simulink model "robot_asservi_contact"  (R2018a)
settings: Solver=VariableStepAuto  StartTime=0.0  StopTime=t(numel(t))  FixedStep=0.0001  RelTol=1e-3
model workspace: external: MATLAB File (data not in the file)
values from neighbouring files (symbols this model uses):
  D = [1500 1500 1000 0 0 0]    [TP_6Axes_main.m]
  dt = 0.01    [TP_6axes_trajectoire_polynomiale.m]    (also in TP_6axes_trajectoire_rectangulaire.m = 0.005)
  I = [0 0 0 0 0 0]    [TP_6Axes_main.m]
  mu = mu/3    [TP_6Axes_main.m]
  nx = length(ref)    [Jnum.m]    (also in TP_6axes_trajectoire_rectangulaire.m = 0.6)
  P = [16000 15000 14000 3000 3000 3000]    [TP_6Axes_main.m]
  q_targ = zeros(6,numel(p_targ(1,:)))    [TP_6axes_trajectoire_polynomiale.m]    (also in TP_6axes_trajectoire_rectangulaire.m)
  X = [T(1:3,4);Euler]    [MGD_6axes.m]    (also in TP_6axes_trajectoire_polynomiale.m = Trace_6axes_trajectoire(q_targ,p_targ,rob); TP_6axes_trajectoire_rectangulaire.m = Trace_6axes_trajectoire(q_targ,p_targ,rob); Trace_6axes.m = [0 0 0; Trace_6axes_trajectoire.m = [0 0 0)
undefined symbols (not defined in the file or in its folder): deg, kg, m, mm, N, rad, s, smiData, Y, Z
libraries: sm_lib x42, nesl_utility x23, Contact_Forces_Lib x1
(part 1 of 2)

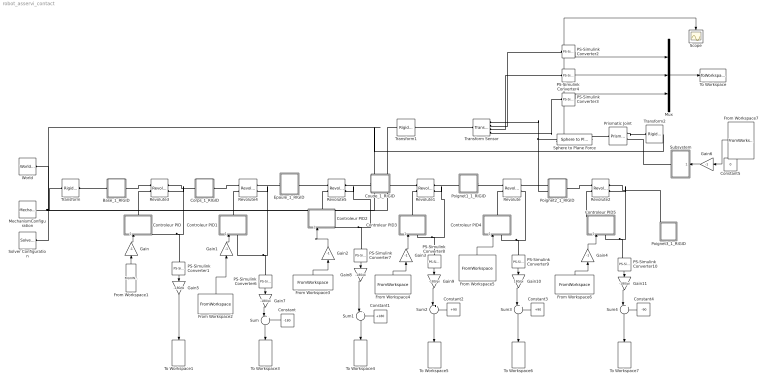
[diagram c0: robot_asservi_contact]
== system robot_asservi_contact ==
  Base_1_RIGID : Subsystem
  Constant : Constant  Value=-180
  Constant1 : Constant  Value=+180
  Constant2 : Constant  Value=+90
  Constant3 : Constant  Value=+90
  Constant4 : Constant  Value=-90
  Constant5 : Constant  Value=0
  Controleur PID : Subsystem
  Controleur PID1 : Subsystem
  Controleur PID2 : Subsystem
  Controleur PID3 : Subsystem
  Controleur PID4 : Subsystem
  Controleur PID5 : Subsystem
  Corps_1_RIGID : Subsystem
  Coude_1_RIGID : Subsystem
  Epaule_1_RIGID : Subsystem
  From Workspace1 : FromWorkspace  VariableName=[t' q_targ(1,:)']  SampleTime=0
  From Workspace2 : FromWorkspace  VariableName=[t' q_targ(2,:)'+pi]  SampleTime=0
  From Workspace3 : FromWorkspace  VariableName=[t' q_targ(3,:)'-pi]  SampleTime=0
  From Workspace4 : FromWorkspace  VariableName=[t' q_targ(4,:)'-pi/2]  SampleTime=0
  From Workspace5 : FromWorkspace  VariableName=[t' q_targ(5,:)'-pi/2]  SampleTime=0
  From Workspace6 : FromWorkspace  VariableName=[t' q_targ(6,:)'+pi/2]  SampleTime=0
  From Workspace7 : FromWorkspace  VariableName=[t' delta'];
  Gain{,1..4,6} (6 alike) : Gain  Gain=-1
  Gain10 : Gain  Gain=180/pi
  Gain{5,7..9,11} (5 alike) : Gain  Gain=-180/pi
  MechanismConfiguration : sm_lib/Utilities/Mechanism Configuration  UniformGravity=None  GravityVector=[0 -9.80665 0]  GravityUnits=m/s^2  LinearizationDelta=0.001
  Mux : Mux  Inputs=3
  PS-Simulink Converter{1,6..10} (6 alike) : nesl_utility/PS-Simulink Converter  PhysicalDomain=network_engine_domain  SubClassName=ps_output  LeftPortType=input  RightPortType=output  PseudoPeriodic=off  Frequencies=[]  Unit=rad  AffineConversion=off
  PS-Simulink Converter2 : nesl_utility/PS-Simulink Converter  PhysicalDomain=network_engine_domain  SubClassName=ps_output  LeftPortType=input  RightPortType=output  PseudoPeriodic=off  Frequencies=[]  Unit=1  AffineConversion=off
  PS-Simulink Converter3 : nesl_utility/PS-Simulink Converter  PhysicalDomain=network_engine_domain  SubClassName=ps_output  LeftPortType=input  RightPortType=output  PseudoPeriodic=off  Frequencies=[]  Unit=1  AffineConversion=off
  PS-Simulink Converter4 : nesl_utility/PS-Simulink Converter  PhysicalDomain=network_engine_domain  SubClassName=ps_output  LeftPortType=input  RightPortType=output  PseudoPeriodic=off  Frequencies=[]  Unit=1  AffineConversion=off
  Poignet1_1_RIGID : Subsystem
  Poignet2_1_RIGID : Subsystem
  Poignet3_1_RIGID : Subsystem
  Prismatic Joint : sm_lib/Joints/Prismatic Joint  SenseConstraintForce=off  SenseConstraintForceX=off  SenseConstraintForceY=off  SenseConstraintForceZ=off  SenseConstraintTorque=off  SenseConstraintTorqueX=off  SenseConstraintTorqueY=off  SenseConstraintTorqueZ=off  SenseTotalForce=off  SenseTotalForceX=off  SenseTotalForceY=off  SenseTotalForceZ=off  SenseTotalTorque=off  SenseTotalTorqueX=off  SenseTotalTorqueY=off  SenseTotalTorqueZ=off  CompositeWrenchDir=FollowerOnBase  CompositeWrenchFrame=BaseFrame  EquilibriumPosition=0  EquilibriumPositionUnits=m  SpringStiffness=0  SpringStiffnessUnits=N/m  DampingCoefficient=0  DampingCoefficientUnits=N/(m/s)  TorqueActuationMode=ComputedTorque  MotionActuationMode=InputMotion  SensePosition=off  SenseVelocity=off  SenseAcceleration=off  SenseTorqueForce=off  PositionTargetSpecify=off  PositionTargetPriority=High  PositionTargetValue=0  PositionTargetValueUnits=m  VelocityTargetSpecify=off  VelocityTargetPriority=High  VelocityTargetValue=0  VelocityTargetValueUnits=m/s
  Revolute : sm_lib/Joints/Revolute Joint  SenseConstraintForce=off  SenseConstraintForceX=off  SenseConstraintForceY=off  SenseConstraintForceZ=off  SenseConstraintTorque=off  SenseConstraintTorqueX=off  SenseConstraintTorqueY=off  SenseConstraintTorqueZ=off  SenseTotalForce=off  SenseTotalForceX=off  SenseTotalForceY=off  SenseTotalForceZ=off  SenseTotalTorque=off  SenseTotalTorqueX=off  SenseTotalTorqueY=off  SenseTotalTorqueZ=off  CompositeWrenchDir=FollowerOnBase  CompositeWrenchFrame=BaseFrame  EquilibriumPosition=0  EquilibriumPositionUnits=rad  SpringStiffness=0  SpringStiffnessUnits=N*m/rad  DampingCoefficient=1/mu(5)  DampingCoefficientUnits=N*m/(rad/s)  TorqueActuationMode=InputTorque  MotionActuationMode=ComputedMotion  SensePosition=on  SenseVelocity=off  SenseAcceleration=off  SenseTorqueForce=off  PositionTargetSpecify=on  PositionTargetPriority=High  PositionTargetValue=q_targ(5,1)-pi/2  PositionTargetValueUnits=rad  VelocityTargetSpecify=off  VelocityTargetPriority=High  VelocityTargetValue=0  VelocityTargetValueUnits=deg/s
  Revolute1 : sm_lib/Joints/Revolute Joint  SenseConstraintForce=off  SenseConstraintForceX=off  SenseConstraintForceY=off  SenseConstraintForceZ=off  SenseConstraintTorque=off  SenseConstraintTorqueX=off  SenseConstraintTorqueY=off  SenseConstraintTorqueZ=off  SenseTotalForce=off  SenseTotalForceX=off  SenseTotalForceY=off  SenseTotalForceZ=off  SenseTotalTorque=off  SenseTotalTorqueX=off  SenseTotalTorqueY=off  SenseTotalTorqueZ=off  CompositeWrenchDir=FollowerOnBase  CompositeWrenchFrame=BaseFrame  EquilibriumPosition=0  EquilibriumPositionUnits=rad  SpringStiffness=0  SpringStiffnessUnits=N*m/rad  DampingCoefficient=1/mu(4)  DampingCoefficientUnits=N*m/(rad/s)  TorqueActuationMode=InputTorque  MotionActuationMode=ComputedMotion  SensePosition=on  SenseVelocity=off  SenseAcceleration=off  SenseTorqueForce=off  PositionTargetSpecify=on  PositionTargetPriority=High  PositionTargetValue=-q_targ(4,1)+pi/2  PositionTargetValueUnits=rad  VelocityTargetSpecify=off  VelocityTargetPriority=High  VelocityTargetValue=0  VelocityTargetValueUnits=deg/s
  Revolute2 : sm_lib/Joints/Revolute Joint  SenseConstraintForce=off  SenseConstraintForceX=off  SenseConstraintForceY=off  SenseConstraintForceZ=off  SenseConstraintTorque=off  SenseConstraintTorqueX=off  SenseConstraintTorqueY=off  SenseConstraintTorqueZ=off  SenseTotalForce=off  SenseTotalForceX=off  SenseTotalForceY=off  SenseTotalForceZ=off  SenseTotalTorque=off  SenseTotalTorqueX=off  SenseTotalTorqueY=off  SenseTotalTorqueZ=off  CompositeWrenchDir=FollowerOnBase  CompositeWrenchFrame=BaseFrame  EquilibriumPosition=0  EquilibriumPositionUnits=rad  SpringStiffness=0  SpringStiffnessUnits=N*m/rad  DampingCoefficient=1/mu(6)  DampingCoefficientUnits=N*m/(rad/s)  TorqueActuationMode=InputTorque  MotionActuationMode=ComputedMotion  SensePosition=on  SenseVelocity=off  SenseAcceleration=off  SenseTorqueForce=off  PositionTargetSpecify=on  PositionTargetPriority=High  PositionTargetValue=-q_targ(6,1)-pi/2  PositionTargetValueUnits=rad  VelocityTargetSpecify=off  VelocityTargetPriority=High  VelocityTargetValue=0  VelocityTargetValueUnits=deg/s
  Revolute3 : sm_lib/Joints/Revolute Joint  SenseConstraintForce=off  SenseConstraintForceX=off  SenseConstraintForceY=off  SenseConstraintForceZ=off  SenseConstraintTorque=off  SenseConstraintTorqueX=off  SenseConstraintTorqueY=off  SenseConstraintTorqueZ=off  SenseTotalForce=off  SenseTotalForceX=off  SenseTotalForceY=off  SenseTotalForceZ=off  SenseTotalTorque=off  SenseTotalTorqueX=off  SenseTotalTorqueY=off  SenseTotalTorqueZ=off  CompositeWrenchDir=FollowerOnBase  CompositeWrenchFrame=BaseFrame  EquilibriumPosition=0  EquilibriumPositionUnits=rad  SpringStiffness=0  SpringStiffnessUnits=N*m/rad  DampingCoefficient=1/mu(1)  DampingCoefficientUnits=N*m/(rad/s)  TorqueActuationMode=InputTorque  MotionActuationMode=ComputedMotion  SensePosition=on  SenseVelocity=off  SenseAcceleration=off  SenseTorqueForce=off  PositionTargetSpecify=on  PositionTargetPriority=High  PositionTargetValue=-q_targ(1,1)  PositionTargetValueUnits=rad  VelocityTargetSpecify=off  VelocityTargetPriority=High  VelocityTargetValue=0  VelocityTargetValueUnits=deg/s
  Revolute4 : sm_lib/Joints/Revolute Joint  SenseConstraintForce=off  SenseConstraintForceX=off  SenseConstraintForceY=off  SenseConstraintForceZ=off  SenseConstraintTorque=off  SenseConstraintTorqueX=off  SenseConstraintTorqueY=off  SenseConstraintTorqueZ=off  SenseTotalForce=off  SenseTotalForceX=off  SenseTotalForceY=off  SenseTotalForceZ=off  SenseTotalTorque=off  SenseTotalTorqueX=off  SenseTotalTorqueY=off  SenseTotalTorqueZ=off  CompositeWrenchDir=FollowerOnBase  CompositeWrenchFrame=BaseFrame  EquilibriumPosition=0  EquilibriumPositionUnits=rad  SpringStiffness=0  SpringStiffnessUnits=N*m/rad  DampingCoefficient=1/mu(2)  DampingCoefficientUnits=N*m/(rad/s)  TorqueActuationMode=InputTorque  MotionActuationMode=ComputedMotion  SensePosition=on  SenseVelocity=off  SenseAcceleration=off  SenseTorqueForce=off  PositionTargetSpecify=on  PositionTargetPriority=High  PositionTargetValue=-q_targ(2,1)-pi  PositionTargetValueUnits=rad  VelocityTargetSpecify=off  VelocityTargetPriority=High  VelocityTargetValue=0  VelocityTargetValueUnits=deg/s
  Revolute5 : sm_lib/Joints/Revolute Joint  SenseConstraintForce=off  SenseConstraintForceX=off  SenseConstraintForceY=off  SenseConstraintForceZ=off  SenseConstraintTorque=off  SenseConstraintTorqueX=off  SenseConstraintTorqueY=off  SenseConstraintTorqueZ=off  SenseTotalForce=off  SenseTotalForceX=off  SenseTotalForceY=off  SenseTotalForceZ=off  SenseTotalTorque=off  SenseTotalTorqueX=off  SenseTotalTorqueY=off  SenseTotalTorqueZ=off  CompositeWrenchDir=FollowerOnBase  CompositeWrenchFrame=BaseFrame  EquilibriumPosition=0  EquilibriumPositionUnits=rad  SpringStiffness=0  SpringStiffnessUnits=N*m/rad  DampingCoefficient=1/mu(3)  DampingCoefficientUnits=N*m/(rad/s)  TorqueActuationMode=InputTorque  MotionActuationMode=ComputedMotion  SensePosition=on  SenseVelocity=off  SenseAcceleration=off  SenseTorqueForce=off  PositionTargetSpecify=on  PositionTargetPriority=High  PositionTargetValue=-q_targ(3,1)+pi  PositionTargetValueUnits=rad  VelocityTargetSpecify=off  VelocityTargetPriority=High  VelocityTargetValue=0  VelocityTargetValueUnits=deg/s
  Scope : Scope
  Solver Configuration : nesl_utility/Solver Configuration  PhysicalDomain=network_engine_domain  SubClassName=solver  LeftPortType=input  RightPortType=generic  Tones=[]  Harmonics=[]  SimulateNoise=off  Profile=off  UseLocalSampling=off  EnableSwitchedLinearOptims=on  FrequencyDomain=off  UseCCode=off  RelTol=0.001  AbsTol=1e-06  MinStep=1e-09  ToWorkspace=off  RevertToSquareIcSolve=off  NumHomotopyIterations=100  PhasorMode=off  PhasorModeNumHarmonics=1  DoDC=off  ResidualTolerance=1e-09  UseLocalSolver=off  LocalSolverChoice=NE_BACKWARD_EULER_ADVANCER  LocalSolverSampleTime=0.001  DoFixedCost=off  MaxNonlinIter=3  MaxModeIter=2  LinearAlgebra=Sparse  EquationFormulation=NE_TIME_EF  DelaysMemoryBudget=1024  AutomaticFiltering=on  FilteringTimeConstant=0.001
  Sphere to Plane Force : Contact_Forces_Lib/3D/Sphere to Plane Force  sphere_rad=e/2  plane_lenx=1  plane_leny=1  plane_depth=e/2  force_law=Nonlinear  k_contact=1e4  b_contact=1e1  pen_full_damp_F=1e-4  pen_exponent=1  custom_param_1=1  custom_param_2=1  friction_law=None  mu_kinetic=0.5  mu_static=0.7  v_thr=0.001  vis_on=on  vis_opc_en=0  vis_len_plaBz=0.005  vis_clr=[0.9 0.2 0.2]  vis_opc=0.7
  Subsystem : Subsystem
  Sum{,1..4} (5 alike) : Sum  Inputs=|++
  To Workspace : ToWorkspace  VariableName=pos_poignet  SaveFormat=Structure  SampleTime=-1
  To Workspace1 : ToWorkspace  VariableName=q_real1  SampleTime=dt
  To Workspace3 : ToWorkspace  VariableName=q_real2  SampleTime=dt
  To Workspace4 : ToWorkspace  VariableName=q_real3  SampleTime=dt
  To Workspace5 : ToWorkspace  VariableName=q_real4  SampleTime=dt
  To Workspace6 : ToWorkspace  VariableName=q_real5  SampleTime=dt
  To Workspace7 : ToWorkspace  VariableName=q_real6  SampleTime=dt
  Transform : sm_lib/Frames and Transforms/Rigid Transform  TranslationMethod=Cartesian  TranslationStandardOffset=0  TranslationLengthUnit=mm  TranslationStandardAxis=+Z  TranslationCartesianOffset=smiData.RigidTransform(10).translation  TranslationROffset=0  TranslationROffsetUnits=m  TranslationZOffset=0  TranslationZOffsetUnits=m  TranslationThetaOffset=0  TranslationThetaOffsetUnits=deg  RotationMethod=ArbitraryAxis  RotationAngleUnits=rad  RotationStandardAxis=+Z  RotationAngle=smiData.RigidTransform(10).angle  RotationArbitraryAxis=smiData.RigidTransform(10).axis  FollAlignAxisA=+X  BaseAlignAxisA=+Y  FollAlignAxisB=+Y  BaseAlignAxisB=+Z  RotationSequenceAxes=FollowerAxes  RotationSequence=XYX  RotationSequenceAngles=[0 0 0]  RotationSequenceAnglesUnits=deg  RotationMatrix=[1 0 0; 0 1 0; 0 0 1]
  Transform Sensor : sm_lib/Frames and Transforms/Transform Sensor  MeasurementFrame=World  SenseAngle=off  SenseAxis=off  SenseAngle1=off  SenseAngle2=off  SenseAngle3=off  SenseQ=off  SenseR=off  SenseOmegaX=off  SenseOmegaY=off  SenseOmegaZ=off  SenseOmega1=off  SenseOmega2=off  SenseOmega3=off  SenseQDot=off  SenseRDot=off  SenseAlphaX=off  SenseAlphaY=off  SenseAlphaZ=off  SenseAlpha1=off  SenseAlpha2=off  SenseAlpha3=off  SenseQDDot=off  SenseRDDot=off  SenseX=on  SenseY=on  SenseZ=on  SenseRad=off  SenseAzim=off  SenseDist=off  SenseInc=off  SenseXDot=off  SenseYDot=off  SenseZDot=off  SenseRadDot=off  SenseAzimDot=off  SenseDistDot=off  SenseIncDot=off  SenseXDDot=off  SenseYDDot=off  SenseZDDot=off  SenseRadDDot=off  SenseAzimDDot=off  SenseDistDDot=off  SenseIncDDot=off
  Transform1 : sm_lib/Frames and Transforms/Rigid Transform  TranslationMethod=StandardAxis  TranslationStandardOffset=350  TranslationLengthUnit=mm  TranslationStandardAxis=+Z  TranslationCartesianOffset=smiData.RigidTransform(10).translation  TranslationROffset=0  TranslationROffsetUnits=m  TranslationZOffset=0  TranslationZOffsetUnits=m  TranslationThetaOffset=0  TranslationThetaOffsetUnits=deg  RotationMethod=None  RotationAngleUnits=rad  RotationStandardAxis=+Z  RotationAngle=smiData.RigidTransform(10).angle  RotationArbitraryAxis=smiData.RigidTransform(10).axis  FollAlignAxisA=+X  BaseAlignAxisA=+Y  FollAlignAxisB=+Y  BaseAlignAxisB=+Z  RotationSequenceAxes=FollowerAxes  RotationSequence=XYX  RotationSequenceAngles=[0 0 0]  RotationSequenceAnglesUnits=deg  RotationMatrix=[1 0 0; 0 1 0; 0 0 1]
  Transform2 : sm_lib/Frames and Transforms/Rigid Transform  TranslationMethod=Cartesian  TranslationStandardOffset=350  TranslationLengthUnit=m  TranslationStandardAxis=+Z  TranslationCartesianOffset=[nx+e/2 0 0.35]  TranslationROffset=0  TranslationROffsetUnits=m  TranslationZOffset=0  TranslationZOffsetUnits=m  TranslationThetaOffset=0  TranslationThetaOffsetUnits=deg  RotationMethod=StandardAxis  RotationAngleUnits=rad  RotationStandardAxis=+Y  RotationAngle=-pi/2  RotationArbitraryAxis=smiData.RigidTransform(10).axis  FollAlignAxisA=+X  BaseAlignAxisA=+Y  FollAlignAxisB=+Y  BaseAlignAxisB=+Z  RotationSequenceAxes=FollowerAxes  RotationSequence=XYX  RotationSequenceAngles=[0 0 0]  RotationSequenceAnglesUnits=deg  RotationMatrix=[1 0 0; 0 1 0; 0 0 1]
  World : sm_lib/Frames and Transforms/World Frame
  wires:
  PS-Simulink Converter2/1 -> Mux/1
  PS-Simulink Converter3/1 -> Mux/3
  PS-Simulink Converter4/1 -> Mux/2
  Mux/1 -> To Workspace/1
  From Workspace2/1 -> Gain1/1
  From Workspace1/1 -> Gain/1
  From Workspace6/1 -> Gain4/1
  Gain/1 -> Controleur PID/1(consigne)
  From Workspace3/1 -> Gain2/1
  Gain1/1 -> Controleur PID1/1(consigne)
  From Workspace4/1 -> Gain3/1
  Gain4/1 -> Controleur PID5/1(consigne)
  From Workspace5/1 -> Controleur PID4/1(consigne)
  Gain2/1 -> Controleur PID2/1(consigne)
  Gain3/1 -> Controleur PID3/1(consigne)
  PS-Simulink Converter1/1 -> Gain5/1
  Gain5/1 -> To Workspace1/1
  PS-Simulink Converter6/1 -> Gain7/1
  PS-Simulink Converter7/1 -> Gain8/1
  PS-Simulink Converter8/1 -> Gain9/1
  PS-Simulink Converter9/1 -> Gain10/1
  PS-Simulink Converter10/1 -> Gain11/1
  Gain7/1 -> Sum/1
  Sum/1 -> To Workspace3/1
  Gain9/1 -> Sum2/1
  Gain11/1 -> Sum4/1
  Gain10/1 -> Sum3/1
  Gain8/1 -> Sum1/1
  Sum1/1 -> To Workspace4/1
  Sum2/1 -> To Workspace5/1
  Sum3/1 -> To Workspace6/1
  Sum4/1 -> To Workspace7/1
  Constant/1 -> Sum/2
  Constant1/1 -> Sum1/2
  Constant2/1 -> Sum2/2
  Constant3/1 -> Sum3/2
  Constant4/1 -> Sum4/2
  Sphere to Plane Force/1 -> Scope/1
  Gain6/1 -> Subsystem/1(In1)
  From Workspace7/1 -> Gain6/1
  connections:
  MechanismConfiguration/RConn1 -- Solver Configuration/RConn1 -- World/RConn1 -- Transform2/LConn1 -- Transform1/LConn1 -- Transform/LConn1
  Poignet1_1_RIGID/RConn1 -- Revolute/LConn1
  Corps_1_RIGID/RConn1 -- Revolute4/LConn1
  Epaule_1_RIGID/LConn1 -- Revolute4/RConn1
  Epaule_1_RIGID/RConn1 -- Revolute5/LConn1
  Coude_1_RIGID/LConn1 -- Revolute5/RConn1
  Poignet2_1_RIGID/LConn1 -- Revolute/RConn1
  Coude_1_RIGID/RConn1 -- Revolute1/LConn1
  Poignet1_1_RIGID/LConn1 -- Revolute1/RConn1
  Poignet2_1_RIGID/RConn1 -- Revolute2/LConn1
  Poignet3_1_RIGID/LConn1 -- Revolute2/RConn1
  Base_1_RIGID/RConn1 -- Revolute3/LConn1
  Corps_1_RIGID/LConn1 -- Revolute3/RConn1
  Base_1_RIGID/LConn1 -- Transform/RConn1
  PS-Simulink Converter3/LConn1 -- Transform Sensor/RConn4
  PS-Simulink Converter2/LConn1 -- Transform Sensor/RConn2
  Poignet2_1_RIGID/LConn2 -- Sphere to Plane Force/LConn1 -- Transform Sensor/RConn1
  Transform1/RConn1 -- Transform Sensor/LConn1
  Transform Sensor/RConn3 -- PS-Simulink Converter4/LConn1
  Controleur PID/RConn1 -- Revolute3/LConn2
  Controleur PID1/RConn1 -- Revolute4/LConn2
  Controleur PID5/RConn1 -- Revolute2/LConn2
  Controleur PID5/LConn1 -- PS-Simulink Converter10/LConn1 -- Revolute2/RConn2
  Controleur PID3/LConn1 -- PS-Simulink Converter8/LConn1 -- Revolute1/RConn2
  Controleur PID4/RConn1 -- Revolute/LConn2
  Controleur PID2/RConn1 -- Revolute5/LConn2
  Controleur PID2/LConn1 -- PS-Simulink Converter7/LConn1 -- Revolute5/RConn2
  Controleur PID3/RConn1 -- Revolute1/LConn2
  Controleur PID1/LConn1 -- PS-Simulink Converter6/LConn1 -- Revolute4/RConn2
  Controleur PID4/LConn1 -- PS-Simulink Converter9/LConn1 -- Revolute/RConn2
  Controleur PID/LConn1 -- PS-Simulink Converter1/LConn1 -- Revolute3/RConn2
  Sphere to Plane Force/RConn1 -- Prismatic Joint/RConn1
  Prismatic Joint/LConn1 -- Transform2/RConn1
  Subsystem/RConn1 -- Prismatic Joint/LConn2

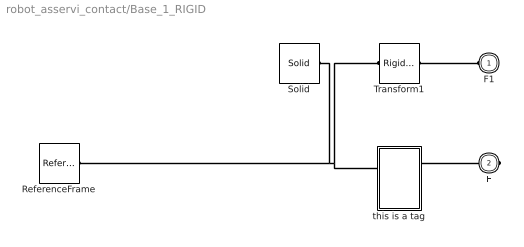
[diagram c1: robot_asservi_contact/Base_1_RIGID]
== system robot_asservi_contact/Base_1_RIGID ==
  ReferenceFrame : sm_lib/Frames and Transforms/Reference Frame
  Solid : sm_lib/Body Elements/Solid  InertiaType=Custom  Mass=smiData.Solid(1).mass  MassUnits=kg  CenterOfMass=smiData.Solid(1).CoM  CenterOfMassUnits=mm  MomentsOfInertia=smiData.Solid(1).MoI  MomentsOfInertiaUnits=kg*mm^2  ProductsOfInertia=smiData.Solid(1).PoI  ProductsOfInertiaUnits=kg*mm^2  DensityBased=on  Density=1000  DensityUnits=kg/m^3  DoExposeReferenceFrame=on  SerializedFrames=<Frames/>  GraphicType=FromGeometry  MarkerShape=Sphere  MarkerSize=10  GraphicVisPropType=SimpleVisualProperties  GraphicDiffuseColor=[1.0 0.0 0.0]  GraphicSpecularColor=[0.5 0.5 0.5 1.0]  GraphicAmbientColor=[0.15 0.15 0.15 1.0]  GraphicEmissiveColor=[0.0 0.0 0.0 1.0]  GraphicShininess=75  GraphicOpacity=smiData.Solid(1).opacity  GeometryShape=FromFile  RectangleSize=[1 1]  RectangleSizeUnits=m  BrickDimensions=[1 1 1]  BrickDimensionUnits=m  CylinderRadius=1  CylinderRadiusUnits=m  CylinderLength=1  CylinderLengthUnits=m  SphereRadius=1  SphereRadiusUnits=m  EllipsoidRadii=[1 1 1]  EllipsoidRadiiUnits=m  ExtrusionCrossSection=[1 1; -1 1; -1 -1; 1 -1]  ExtrusionCrossSectionUnits=m  ExtrusionLength=1  ExtrusionLengthUnits=m  PolygonNumSides=3  PolygonOuterRadius=1  PolygonOuterRadiusUnits=m  ExtGeomFileType=STL  ExtGeomFileName=Base_Défaut_sldprt.STL  ExtGeomFileUnits=mm  RevolutionCrossSection=[1 1; 1 -1; 2 -1; 2 1]  RevolutionCrossSectionUnits=m  RevolutionExtent=Full  RevolutionAngle=180  RevolutionAngleUnits=deg
  Transform1 : sm_lib/Frames and Transforms/Rigid Transform  TranslationMethod=Cartesian  TranslationStandardOffset=0  TranslationLengthUnit=mm  TranslationStandardAxis=+Z  TranslationCartesianOffset=smiData.RigidTransform(9).translation  TranslationROffset=0  TranslationROffsetUnits=m  TranslationZOffset=0  TranslationZOffsetUnits=m  TranslationThetaOffset=0  TranslationThetaOffsetUnits=deg  RotationMethod=ArbitraryAxis  RotationAngleUnits=rad  RotationStandardAxis=+Z  RotationAngle=smiData.RigidTransform(9).angle  RotationArbitraryAxis=smiData.RigidTransform(9).axis  FollAlignAxisA=+X  BaseAlignAxisA=+Y  FollAlignAxisB=+Y  BaseAlignAxisB=+Z  RotationSequenceAxes=FollowerAxes  RotationSequence=XYX  RotationSequenceAngles=[0 0 0]  RotationSequenceAnglesUnits=deg  RotationMatrix=[1 0 0; 0 1 0; 0 0 1]
  this is a tag : Subsystem
  F1 : PMIOPort  Side=Left
  F : PMIOPort  Port=2  Side=Right
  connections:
  Transform1/RConn1 -- F1/RConn1
  ReferenceFrame/RConn1 -- Solid/RConn1 -- this is a tag/LConn1 -- Transform1/LConn1
  this is a tag/RConn1 -- F/RConn1

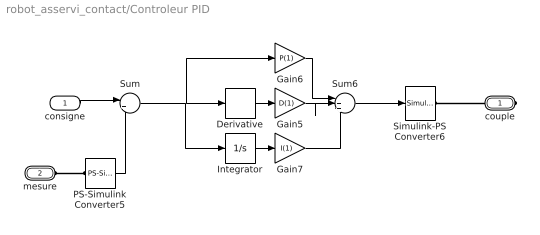
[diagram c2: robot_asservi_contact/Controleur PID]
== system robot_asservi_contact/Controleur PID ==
  consigne : Inport
  Derivative : Derivative
  Gain5 : Gain  Gain=D(1)
  Gain6 : Gain  Gain=P(1)
  Gain7 : Gain  Gain=I(1)
  Integrator : Integrator
  PS-Simulink Converter5 : nesl_utility/PS-Simulink Converter  PhysicalDomain=network_engine_domain  SubClassName=ps_output  LeftPortType=input  RightPortType=output  PseudoPeriodic=off  Frequencies=[]  Unit=rad  AffineConversion=off
  Simulink-PS Converter6 : nesl_utility/Simulink-PS Converter  PhysicalDomain=network_engine_domain  SubClassName=ps_input  LeftPortType=input  RightPortType=output  PseudoPeriodic=off  Frequencies=[]  NoiseDistribution=none  NoiseParameters=[]  Unit=N*m  AffineConversion=off  FilteringAndDerivatives=zero  SimscapeFilterOrder=1  InputFilterTimeConstant=0.001  UdotUserProvided=2
  Sum : Sum  Inputs=|+-
  Sum6 : Sum  Inputs=|+++
  couple : PMIOPort  Side=Right
  mesure : PMIOPort  Port=2  Side=Left
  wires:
  Gain7/1 -> Sum6/3
  Gain5/1 -> Sum6/2
  Derivative/1 -> Gain5/1
  Sum6/1 -> Simulink-PS Converter6/1
  Gain6/1 -> Sum6/1
  Integrator/1 -> Gain7/1
  consigne/1 -> Sum/1
  PS-Simulink Converter5/1 -> Sum/2
  Sum/1 -> Integrator/1, Gain6/1, Derivative/1
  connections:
  Simulink-PS Converter6/RConn1 -- couple/RConn1
  mesure/RConn1 -- PS-Simulink Converter5/LConn1

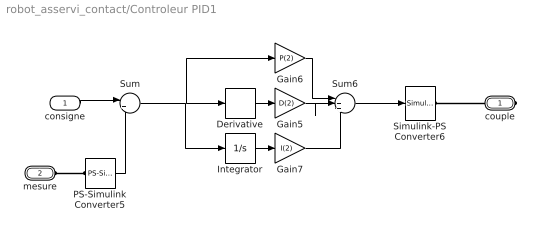
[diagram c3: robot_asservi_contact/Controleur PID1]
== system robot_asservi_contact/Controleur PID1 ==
  consigne : Inport
  Derivative : Derivative
  Gain5 : Gain  Gain=D(2)
  Gain6 : Gain  Gain=P(2)
  Gain7 : Gain  Gain=I(2)
  Integrator : Integrator
  PS-Simulink Converter5 : nesl_utility/PS-Simulink Converter  PhysicalDomain=network_engine_domain  SubClassName=ps_output  LeftPortType=input  RightPortType=output  PseudoPeriodic=off  Frequencies=[]  Unit=rad  AffineConversion=off
  Simulink-PS Converter6 : nesl_utility/Simulink-PS Converter  PhysicalDomain=network_engine_domain  SubClassName=ps_input  LeftPortType=input  RightPortType=output  PseudoPeriodic=off  Frequencies=[]  NoiseDistribution=none  NoiseParameters=[]  Unit=N*m  AffineConversion=off  FilteringAndDerivatives=zero  SimscapeFilterOrder=1  InputFilterTimeConstant=0.001  UdotUserProvided=2
  Sum : Sum  Inputs=|+-
  Sum6 : Sum  Inputs=|+++
  couple : PMIOPort  Side=Right
  mesure : PMIOPort  Port=2  Side=Left
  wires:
  Gain7/1 -> Sum6/3
  Gain5/1 -> Sum6/2
  Derivative/1 -> Gain5/1
  Sum6/1 -> Simulink-PS Converter6/1
  Gain6/1 -> Sum6/1
  Integrator/1 -> Gain7/1
  consigne/1 -> Sum/1
  PS-Simulink Converter5/1 -> Sum/2
  Sum/1 -> Integrator/1, Gain6/1, Derivative/1
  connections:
  Simulink-PS Converter6/RConn1 -- couple/RConn1
  mesure/RConn1 -- PS-Simulink Converter5/LConn1

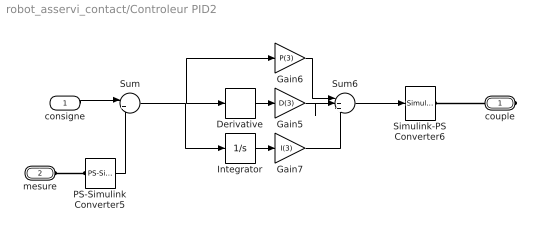
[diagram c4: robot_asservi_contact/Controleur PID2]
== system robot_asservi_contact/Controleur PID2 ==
  consigne : Inport
  Derivative : Derivative
  Gain5 : Gain  Gain=D(3)
  Gain6 : Gain  Gain=P(3)
  Gain7 : Gain  Gain=I(3)
  Integrator : Integrator
  PS-Simulink Converter5 : nesl_utility/PS-Simulink Converter  PhysicalDomain=network_engine_domain  SubClassName=ps_output  LeftPortType=input  RightPortType=output  PseudoPeriodic=off  Frequencies=[]  Unit=rad  AffineConversion=off
  Simulink-PS Converter6 : nesl_utility/Simulink-PS Converter  PhysicalDomain=network_engine_domain  SubClassName=ps_input  LeftPortType=input  RightPortType=output  PseudoPeriodic=off  Frequencies=[]  NoiseDistribution=none  NoiseParameters=[]  Unit=N*m  AffineConversion=off  FilteringAndDerivatives=zero  SimscapeFilterOrder=1  InputFilterTimeConstant=0.001  UdotUserProvided=2
  Sum : Sum  Inputs=|+-
  Sum6 : Sum  Inputs=|+++
  couple : PMIOPort  Side=Right
  mesure : PMIOPort  Port=2  Side=Left
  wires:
  Gain7/1 -> Sum6/3
  Gain5/1 -> Sum6/2
  Derivative/1 -> Gain5/1
  Sum6/1 -> Simulink-PS Converter6/1
  Gain6/1 -> Sum6/1
  Integrator/1 -> Gain7/1
  consigne/1 -> Sum/1
  PS-Simulink Converter5/1 -> Sum/2
  Sum/1 -> Integrator/1, Gain6/1, Derivative/1
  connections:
  Simulink-PS Converter6/RConn1 -- couple/RConn1
  mesure/RConn1 -- PS-Simulink Converter5/LConn1

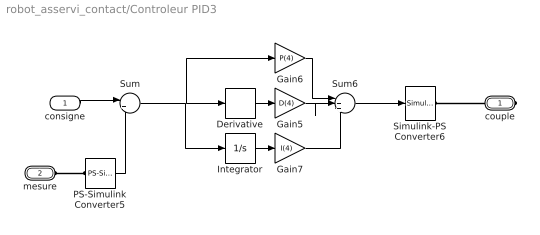
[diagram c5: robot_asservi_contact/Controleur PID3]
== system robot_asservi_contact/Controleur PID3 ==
  consigne : Inport
  Derivative : Derivative
  Gain5 : Gain  Gain=D(4)
  Gain6 : Gain  Gain=P(4)
  Gain7 : Gain  Gain=I(4)
  Integrator : Integrator
  PS-Simulink Converter5 : nesl_utility/PS-Simulink Converter  PhysicalDomain=network_engine_domain  SubClassName=ps_output  LeftPortType=input  RightPortType=output  PseudoPeriodic=off  Frequencies=[]  Unit=rad  AffineConversion=off
  Simulink-PS Converter6 : nesl_utility/Simulink-PS Converter  PhysicalDomain=network_engine_domain  SubClassName=ps_input  LeftPortType=input  RightPortType=output  PseudoPeriodic=off  Frequencies=[]  NoiseDistribution=none  NoiseParameters=[]  Unit=N*m  AffineConversion=off  FilteringAndDerivatives=zero  SimscapeFilterOrder=1  InputFilterTimeConstant=0.001  UdotUserProvided=2
  Sum : Sum  Inputs=|+-
  Sum6 : Sum  Inputs=|+++
  couple : PMIOPort  Side=Right
  mesure : PMIOPort  Port=2  Side=Left
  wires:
  Gain7/1 -> Sum6/3
  Gain5/1 -> Sum6/2
  Derivative/1 -> Gain5/1
  Sum6/1 -> Simulink-PS Converter6/1
  Gain6/1 -> Sum6/1
  Integrator/1 -> Gain7/1
  consigne/1 -> Sum/1
  PS-Simulink Converter5/1 -> Sum/2
  Sum/1 -> Integrator/1, Gain6/1, Derivative/1
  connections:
  Simulink-PS Converter6/RConn1 -- couple/RConn1
  mesure/RConn1 -- PS-Simulink Converter5/LConn1

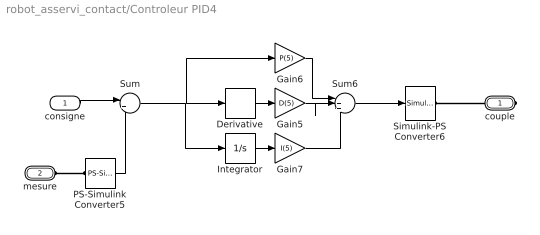
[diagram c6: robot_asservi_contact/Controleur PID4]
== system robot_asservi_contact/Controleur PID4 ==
  consigne : Inport
  Derivative : Derivative
  Gain5 : Gain  Gain=D(5)
  Gain6 : Gain  Gain=P(5)
  Gain7 : Gain  Gain=I(5)
  Integrator : Integrator
  PS-Simulink Converter5 : nesl_utility/PS-Simulink Converter  PhysicalDomain=network_engine_domain  SubClassName=ps_output  LeftPortType=input  RightPortType=output  PseudoPeriodic=off  Frequencies=[]  Unit=rad  AffineConversion=off
  Simulink-PS Converter6 : nesl_utility/Simulink-PS Converter  PhysicalDomain=network_engine_domain  SubClassName=ps_input  LeftPortType=input  RightPortType=output  PseudoPeriodic=off  Frequencies=[]  NoiseDistribution=none  NoiseParameters=[]  Unit=N*m  AffineConversion=off  FilteringAndDerivatives=zero  SimscapeFilterOrder=1  InputFilterTimeConstant=0.001  UdotUserProvided=2
  Sum : Sum  Inputs=|+-
  Sum6 : Sum  Inputs=|+++
  couple : PMIOPort  Side=Right
  mesure : PMIOPort  Port=2  Side=Left
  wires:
  Gain7/1 -> Sum6/3
  Gain5/1 -> Sum6/2
  Derivative/1 -> Gain5/1
  Sum6/1 -> Simulink-PS Converter6/1
  Gain6/1 -> Sum6/1
  Integrator/1 -> Gain7/1
  consigne/1 -> Sum/1
  PS-Simulink Converter5/1 -> Sum/2
  Sum/1 -> Integrator/1, Gain6/1, Derivative/1
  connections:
  Simulink-PS Converter6/RConn1 -- couple/RConn1
  mesure/RConn1 -- PS-Simulink Converter5/LConn1

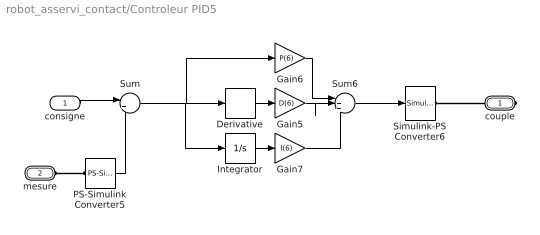
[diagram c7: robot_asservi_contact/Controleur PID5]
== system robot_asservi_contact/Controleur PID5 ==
  consigne : Inport
  Derivative : Derivative
  Gain5 : Gain  Gain=D(6)
  Gain6 : Gain  Gain=P(6)
  Gain7 : Gain  Gain=I(6)
  Integrator : Integrator
  PS-Simulink Converter5 : nesl_utility/PS-Simulink Converter  PhysicalDomain=network_engine_domain  SubClassName=ps_output  LeftPortType=input  RightPortType=output  PseudoPeriodic=off  Frequencies=[]  Unit=rad  AffineConversion=off
  Simulink-PS Converter6 : nesl_utility/Simulink-PS Converter  PhysicalDomain=network_engine_domain  SubClassName=ps_input  LeftPortType=input  RightPortType=output  PseudoPeriodic=off  Frequencies=[]  NoiseDistribution=none  NoiseParameters=[]  Unit=N*m  AffineConversion=off  FilteringAndDerivatives=zero  SimscapeFilterOrder=1  InputFilterTimeConstant=0.001  UdotUserProvided=2
  Sum : Sum  Inputs=|+-
  Sum6 : Sum  Inputs=|+++
  couple : PMIOPort  Side=Right
  mesure : PMIOPort  Port=2  Side=Left
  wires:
  Gain7/1 -> Sum6/3
  Gain5/1 -> Sum6/2
  Derivative/1 -> Gain5/1
  Sum6/1 -> Simulink-PS Converter6/1
  Gain6/1 -> Sum6/1
  Integrator/1 -> Gain7/1
  consigne/1 -> Sum/1
  PS-Simulink Converter5/1 -> Sum/2
  Sum/1 -> Integrator/1, Gain6/1, Derivative/1
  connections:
  Simulink-PS Converter6/RConn1 -- couple/RConn1
  mesure/RConn1 -- PS-Simulink Converter5/LConn1

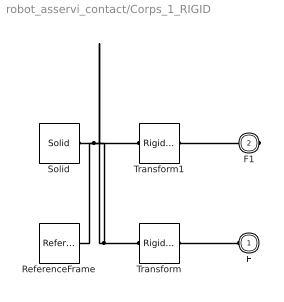
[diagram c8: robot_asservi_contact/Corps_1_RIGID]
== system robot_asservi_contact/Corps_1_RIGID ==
  ReferenceFrame : sm_lib/Frames and Transforms/Reference Frame
  Solid : sm_lib/Body Elements/Solid  InertiaType=Custom  Mass=smiData.Solid(3).mass  MassUnits=kg  CenterOfMass=smiData.Solid(3).CoM  CenterOfMassUnits=mm  MomentsOfInertia=smiData.Solid(3).MoI  MomentsOfInertiaUnits=kg*mm^2  ProductsOfInertia=smiData.Solid(3).PoI  ProductsOfInertiaUnits=kg*mm^2  DensityBased=on  Density=1000  DensityUnits=kg/m^3  DoExposeReferenceFrame=on  SerializedFrames=<Frames/>  GraphicType=FromGeometry  MarkerShape=Sphere  MarkerSize=10  GraphicVisPropType=SimpleVisualProperties  GraphicDiffuseColor=[0.4 1.0 0.6]  GraphicSpecularColor=[0.5 0.5 0.5 1.0]  GraphicAmbientColor=[0.15 0.15 0.15 1.0]  GraphicEmissiveColor=[0.0 0.0 0.0 1.0]  GraphicShininess=75  GraphicOpacity=smiData.Solid(3).opacity  GeometryShape=FromFile  RectangleSize=[1 1]  RectangleSizeUnits=m  BrickDimensions=[1 1 1]  BrickDimensionUnits=m  CylinderRadius=1  CylinderRadiusUnits=m  CylinderLength=1  CylinderLengthUnits=m  SphereRadius=1  SphereRadiusUnits=m  EllipsoidRadii=[1 1 1]  EllipsoidRadiiUnits=m  ExtrusionCrossSection=[1 1; -1 1; -1 -1; 1 -1]  ExtrusionCrossSectionUnits=m  ExtrusionLength=1  ExtrusionLengthUnits=m  PolygonNumSides=3  PolygonOuterRadius=1  PolygonOuterRadiusUnits=m  ExtGeomFileType=STL  ExtGeomFileName=Corps_Défaut_sldprt.STL  ExtGeomFileUnits=mm  RevolutionCrossSection=[1 1; 1 -1; 2 -1; 2 1]  RevolutionCrossSectionUnits=m  RevolutionExtent=Full  RevolutionAngle=180  RevolutionAngleUnits=deg
  Transform : sm_lib/Frames and Transforms/Rigid Transform  TranslationMethod=Cartesian  TranslationStandardOffset=0  TranslationLengthUnit=mm  TranslationStandardAxis=+Z  TranslationCartesianOffset=smiData.RigidTransform(8).translation  TranslationROffset=0  TranslationROffsetUnits=m  TranslationZOffset=0  TranslationZOffsetUnits=m  TranslationThetaOffset=0  TranslationThetaOffsetUnits=deg  RotationMethod=ArbitraryAxis  RotationAngleUnits=rad  RotationStandardAxis=+Z  RotationAngle=smiData.RigidTransform(8).angle  RotationArbitraryAxis=smiData.RigidTransform(8).axis  FollAlignAxisA=+X  BaseAlignAxisA=+Y  FollAlignAxisB=+Y  BaseAlignAxisB=+Z  RotationSequenceAxes=FollowerAxes  RotationSequence=XYX  RotationSequenceAngles=[0 0 0]  RotationSequenceAnglesUnits=deg  RotationMatrix=[1 0 0; 0 1 0; 0 0 1]
  Transform1 : sm_lib/Frames and Transforms/Rigid Transform  TranslationMethod=Cartesian  TranslationStandardOffset=0  TranslationLengthUnit=mm  TranslationStandardAxis=+Z  TranslationCartesianOffset=smiData.RigidTransform(11).translation  TranslationROffset=0  TranslationROffsetUnits=m  TranslationZOffset=0  TranslationZOffsetUnits=m  TranslationThetaOffset=0  TranslationThetaOffsetUnits=deg  RotationMethod=ArbitraryAxis  RotationAngleUnits=rad  RotationStandardAxis=+Z  RotationAngle=smiData.RigidTransform(11).angle  RotationArbitraryAxis=smiData.RigidTransform(11).axis  FollAlignAxisA=+X  BaseAlignAxisA=+Y  FollAlignAxisB=+Y  BaseAlignAxisB=+Z  RotationSequenceAxes=FollowerAxes  RotationSequence=XYX  RotationSequenceAngles=[0 0 0]  RotationSequenceAnglesUnits=deg  RotationMatrix=[1 0 0; 0 1 0; 0 0 1]
  F : PMIOPort  Side=Left
  F1 : PMIOPort  Port=2  Side=Right
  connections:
  Solid/RConn1 -- ReferenceFrame/RConn1 -- Transform/LConn1 -- Transform1/LConn1
  Transform/RConn1 -- F/RConn1
  Transform1/RConn1 -- F1/RConn1

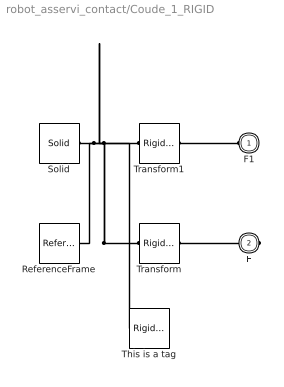
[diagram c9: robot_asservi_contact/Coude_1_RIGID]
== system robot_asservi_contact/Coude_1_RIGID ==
  ReferenceFrame : sm_lib/Frames and Transforms/Reference Frame
  Solid : sm_lib/Body Elements/Solid  InertiaType=Custom  Mass=smiData.Solid(4).mass  MassUnits=kg  CenterOfMass=smiData.Solid(4).CoM  CenterOfMassUnits=mm  MomentsOfInertia=smiData.Solid(4).MoI  MomentsOfInertiaUnits=kg*mm^2  ProductsOfInertia=smiData.Solid(4).PoI  ProductsOfInertiaUnits=kg*mm^2  DensityBased=on  Density=1000  DensityUnits=kg/m^3  DoExposeReferenceFrame=on  SerializedFrames=<Frames/>  GraphicType=FromGeometry  MarkerShape=Sphere  MarkerSize=10  GraphicVisPropType=SimpleVisualProperties  GraphicDiffuseColor=[0.4 0.8 1.0]  GraphicSpecularColor=[0.5 0.5 0.5 1.0]  GraphicAmbientColor=[0.15 0.15 0.15 1.0]  GraphicEmissiveColor=[0.0 0.0 0.0 1.0]  GraphicShininess=75  GraphicOpacity=smiData.Solid(4).opacity  GeometryShape=FromFile  RectangleSize=[1 1]  RectangleSizeUnits=m  BrickDimensions=[1 1 1]  BrickDimensionUnits=m  CylinderRadius=1  CylinderRadiusUnits=m  CylinderLength=1  CylinderLengthUnits=m  SphereRadius=1  SphereRadiusUnits=m  EllipsoidRadii=[1 1 1]  EllipsoidRadiiUnits=m  ExtrusionCrossSection=[1 1; -1 1; -1 -1; 1 -1]  ExtrusionCrossSectionUnits=m  ExtrusionLength=1  ExtrusionLengthUnits=m  PolygonNumSides=3  PolygonOuterRadius=1  PolygonOuterRadiusUnits=m  ExtGeomFileType=STL  ExtGeomFileName=Coude_Défaut_sldprt.STL  ExtGeomFileUnits=mm  RevolutionCrossSection=[1 1; 1 -1; 2 -1; 2 1]  RevolutionCrossSectionUnits=m  RevolutionExtent=Full  RevolutionAngle=180  RevolutionAngleUnits=deg
  This is a tag : sm_lib/Frames and Transforms/Rigid Transform  TranslationMethod=Cartesian  TranslationStandardOffset=0  TranslationLengthUnit=mm  TranslationStandardAxis=+Z  TranslationCartesianOffset=smiData.RigidTransform(3).translation  TranslationROffset=0  TranslationROffsetUnits=m  TranslationZOffset=0  TranslationZOffsetUnits=m  TranslationThetaOffset=0  TranslationThetaOffsetUnits=deg  RotationMethod=ArbitraryAxis  RotationAngleUnits=rad  RotationStandardAxis=+Z  RotationAngle=smiData.RigidTransform(3).angle  RotationArbitraryAxis=smiData.RigidTransform(3).axis  FollAlignAxisA=+X  BaseAlignAxisA=+Y  FollAlignAxisB=+Y  BaseAlignAxisB=+Z  RotationSequenceAxes=FollowerAxes  RotationSequence=XYX  RotationSequenceAngles=[0 0 0]  RotationSequenceAnglesUnits=deg  RotationMatrix=[1 0 0; 0 1 0; 0 0 1]
  Transform : sm_lib/Frames and Transforms/Rigid Transform  TranslationMethod=Cartesian  TranslationStandardOffset=0  TranslationLengthUnit=mm  TranslationStandardAxis=+Z  TranslationCartesianOffset=smiData.RigidTransform(3).translation  TranslationROffset=0  TranslationROffsetUnits=m  TranslationZOffset=0  TranslationZOffsetUnits=m  TranslationThetaOffset=0  TranslationThetaOffsetUnits=deg  RotationMethod=ArbitraryAxis  RotationAngleUnits=rad  RotationStandardAxis=+Z  RotationAngle=smiData.RigidTransform(3).angle  RotationArbitraryAxis=smiData.RigidTransform(3).axis  FollAlignAxisA=+X  BaseAlignAxisA=+Y  FollAlignAxisB=+Y  BaseAlignAxisB=+Z  RotationSequenceAxes=FollowerAxes  RotationSequence=XYX  RotationSequenceAngles=[0 0 0]  RotationSequenceAnglesUnits=deg  RotationMatrix=[1 0 0; 0 1 0; 0 0 1]
  Transform1 : sm_lib/Frames and Transforms/Rigid Transform  TranslationMethod=Cartesian  TranslationStandardOffset=0  TranslationLengthUnit=mm  TranslationStandardAxis=+Z  TranslationCartesianOffset=smiData.RigidTransform(14).translation  TranslationROffset=0  TranslationROffsetUnits=m  TranslationZOffset=0  TranslationZOffsetUnits=m  TranslationThetaOffset=0  TranslationThetaOffsetUnits=deg  RotationMethod=ArbitraryAxis  RotationAngleUnits=rad  RotationStandardAxis=+Z  RotationAngle=smiData.RigidTransform(14).angle  RotationArbitraryAxis=smiData.RigidTransform(14).axis  FollAlignAxisA=+X  BaseAlignAxisA=+Y  FollAlignAxisB=+Y  BaseAlignAxisB=+Z  RotationSequenceAxes=FollowerAxes  RotationSequence=XYX  RotationSequenceAngles=[0 0 0]  RotationSequenceAnglesUnits=deg  RotationMatrix=[1 0 0; 0 1 0; 0 0 1]
  F1 : PMIOPort  Side=Left
  F : PMIOPort  Port=2  Side=Right
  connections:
  Solid/RConn1 -- ReferenceFrame/RConn1 -- This is a tag/LConn1 -- Transform/LConn1 -- Transform1/LConn1
  Transform/RConn1 -- F/RConn1
  Transform1/RConn1 -- F1/RConn1

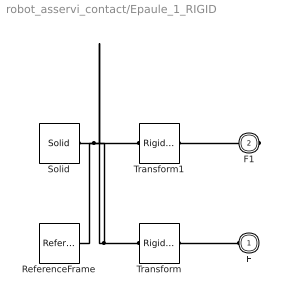
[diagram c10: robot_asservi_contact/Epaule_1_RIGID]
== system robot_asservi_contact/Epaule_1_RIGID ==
  ReferenceFrame : sm_lib/Frames and Transforms/Reference Frame
  Solid : sm_lib/Body Elements/Solid  InertiaType=Custom  Mass=smiData.Solid(7).mass  MassUnits=kg  CenterOfMass=smiData.Solid(7).CoM  CenterOfMassUnits=mm  MomentsOfInertia=smiData.Solid(7).MoI  MomentsOfInertiaUnits=kg*mm^2  ProductsOfInertia=smiData.Solid(7).PoI  ProductsOfInertiaUnits=kg*mm^2  DensityBased=on  Density=1000  DensityUnits=kg/m^3  DoExposeReferenceFrame=on  SerializedFrames=<Frames/>  GraphicType=FromGeometry  MarkerShape=Sphere  MarkerSize=10  GraphicVisPropType=SimpleVisualProperties  GraphicDiffuseColor=[1.0 0.6 0.4]  GraphicSpecularColor=[0.5 0.5 0.5 1.0]  GraphicAmbientColor=[0.15 0.15 0.15 1.0]  GraphicEmissiveColor=[0.0 0.0 0.0 1.0]  GraphicShininess=75  GraphicOpacity=smiData.Solid(7).opacity  GeometryShape=FromFile  RectangleSize=[1 1]  RectangleSizeUnits=m  BrickDimensions=[1 1 1]  BrickDimensionUnits=m  CylinderRadius=1  CylinderRadiusUnits=m  CylinderLength=1  CylinderLengthUnits=m  SphereRadius=1  SphereRadiusUnits=m  EllipsoidRadii=[1 1 1]  EllipsoidRadiiUnits=m  ExtrusionCrossSection=[1 1; -1 1; -1 -1; 1 -1]  ExtrusionCrossSectionUnits=m  ExtrusionLength=1  ExtrusionLengthUnits=m  PolygonNumSides=3  PolygonOuterRadius=1  PolygonOuterRadiusUnits=m  ExtGeomFileType=STL  ExtGeomFileName=Epaule_Défaut_sldprt.STL  ExtGeomFileUnits=mm  RevolutionCrossSection=[1 1; 1 -1; 2 -1; 2 1]  RevolutionCrossSectionUnits=m  RevolutionExtent=Full  RevolutionAngle=180  RevolutionAngleUnits=deg
  Transform : sm_lib/Frames and Transforms/Rigid Transform  TranslationMethod=Cartesian  TranslationStandardOffset=0  TranslationLengthUnit=mm  TranslationStandardAxis=+Z  TranslationCartesianOffset=smiData.RigidTransform(12).translation  TranslationROffset=0  TranslationROffsetUnits=m  TranslationZOffset=0  TranslationZOffsetUnits=m  TranslationThetaOffset=0  TranslationThetaOffsetUnits=deg  RotationMethod=ArbitraryAxis  RotationAngleUnits=rad  RotationStandardAxis=+Z  RotationAngle=smiData.RigidTransform(12).angle  RotationArbitraryAxis=smiData.RigidTransform(12).axis  FollAlignAxisA=+X  BaseAlignAxisA=+Y  FollAlignAxisB=+Y  BaseAlignAxisB=+Z  RotationSequenceAxes=FollowerAxes  RotationSequence=XYX  RotationSequenceAngles=[0 0 0]  RotationSequenceAnglesUnits=deg  RotationMatrix=[1 0 0; 0 1 0; 0 0 1]
  Transform1 : sm_lib/Frames and Transforms/Rigid Transform  TranslationMethod=Cartesian  TranslationStandardOffset=0  TranslationLengthUnit=mm  TranslationStandardAxis=+Z  TranslationCartesianOffset=smiData.RigidTransform(13).translation  TranslationROffset=0  TranslationROffsetUnits=m  TranslationZOffset=0  TranslationZOffsetUnits=m  TranslationThetaOffset=0  TranslationThetaOffsetUnits=deg  RotationMethod=ArbitraryAxis  RotationAngleUnits=rad  RotationStandardAxis=+Z  RotationAngle=smiData.RigidTransform(13).angle  RotationArbitraryAxis=smiData.RigidTransform(13).axis  FollAlignAxisA=+X  BaseAlignAxisA=+Y  FollAlignAxisB=+Y  BaseAlignAxisB=+Z  RotationSequenceAxes=FollowerAxes  RotationSequence=XYX  RotationSequenceAngles=[0 0 0]  RotationSequenceAnglesUnits=deg  RotationMatrix=[1 0 0; 0 1 0; 0 0 1]
  F : PMIOPort  Side=Left
  F1 : PMIOPort  Port=2  Side=Right
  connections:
  Solid/RConn1 -- ReferenceFrame/RConn1 -- Transform/LConn1 -- Transform1/LConn1
  Transform/RConn1 -- F/RConn1
  Transform1/RConn1 -- F1/RConn1

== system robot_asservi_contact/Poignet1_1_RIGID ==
  ReferenceFrame : sm_lib/Frames and Transforms/Reference Frame
  Solid : sm_lib/Body Elements/Solid  InertiaType=Custom  Mass=smiData.Solid(5).mass  MassUnits=kg  CenterOfMass=smiData.Solid(5).CoM  CenterOfMassUnits=mm  MomentsOfInertia=smiData.Solid(5).MoI  MomentsOfInertiaUnits=kg*mm^2  ProductsOfInertia=smiData.Solid(5).PoI  ProductsOfInertiaUnits=kg*mm^2  DensityBased=on  Density=1000  DensityUnits=kg/m^3  DoExposeReferenceFrame=on  SerializedFrames=<Frames/>  GraphicType=FromGeometry  MarkerShape=Sphere  MarkerSize=10  GraphicVisPropType=SimpleVisualProperties  GraphicDiffuseColor=[0.6 0.6 1.0]  GraphicSpecularColor=[0.5 0.5 0.5 1.0]  GraphicAmbientColor=[0.15 0.15 0.15 1.0]  GraphicEmissiveColor=[0.0 0.0 0.0 1.0]  GraphicShininess=75  GraphicOpacity=smiData.Solid(5).opacity  GeometryShape=FromFile  RectangleSize=[1 1]  RectangleSizeUnits=m  BrickDimensions=[1 1 1]  BrickDimensionUnits=m  CylinderRadius=1  CylinderRadiusUnits=m  CylinderLength=1  CylinderLengthUnits=m  SphereRadius=1  SphereRadiusUnits=m  EllipsoidRadii=[1 1 1]  EllipsoidRadiiUnits=m  ExtrusionCrossSection=[1 1; -1 1; -1 -1; 1 -1]  ExtrusionCrossSectionUnits=m  ExtrusionLength=1  ExtrusionLengthUnits=m  PolygonNumSides=3  PolygonOuterRadius=1  PolygonOuterRadiusUnits=m  ExtGeomFileType=STL  ExtGeomFileName=Poignet1_Défaut_sldprt.STL  ExtGeomFileUnits=mm  RevolutionCrossSection=[1 1; 1 -1; 2 -1; 2 1]  RevolutionCrossSectionUnits=m  RevolutionExtent=Full  RevolutionAngle=180  RevolutionAngleUnits=deg
  Transform : sm_lib/Frames and Transforms/Rigid Transform  TranslationMethod=Cartesian  TranslationStandardOffset=0  TranslationLengthUnit=mm  TranslationStandardAxis=+Z  TranslationCartesianOffset=smiData.RigidTransform(1).translation  TranslationROffset=0  TranslationROffsetUnits=m  TranslationZOffset=0  TranslationZOffsetUnits=m  TranslationThetaOffset=0  TranslationThetaOffsetUnits=deg  RotationMethod=ArbitraryAxis  RotationAngleUnits=rad  RotationStandardAxis=+Z  RotationAngle=smiData.RigidTransform(1).angle  RotationArbitraryAxis=smiData.RigidTransform(1).axis  FollAlignAxisA=+X  BaseAlignAxisA=+Y  FollAlignAxisB=+Y  BaseAlignAxisB=+Z  RotationSequenceAxes=FollowerAxes  RotationSequence=XYX  RotationSequenceAngles=[0 0 0]  RotationSequenceAnglesUnits=deg  RotationMatrix=[1 0 0; 0 1 0; 0 0 1]
  Transform1 : sm_lib/Frames and Transforms/Rigid Transform  TranslationMethod=Cartesian  TranslationStandardOffset=0  TranslationLengthUnit=mm  TranslationStandardAxis=+Z  TranslationCartesianOffset=smiData.RigidTransform(4).translation  TranslationROffset=0  TranslationROffsetUnits=m  TranslationZOffset=0  TranslationZOffsetUnits=m  TranslationThetaOffset=0  TranslationThetaOffsetUnits=deg  RotationMethod=ArbitraryAxis  RotationAngleUnits=rad  RotationStandardAxis=+Z  RotationAngle=smiData.RigidTransform(4).angle  RotationArbitraryAxis=smiData.RigidTransform(4).axis  FollAlignAxisA=+X  BaseAlignAxisA=+Y  FollAlignAxisB=+Y  BaseAlignAxisB=+Z  RotationSequenceAxes=FollowerAxes  RotationSequence=XYX  RotationSequenceAngles=[0 0 0]  RotationSequenceAnglesUnits=deg  RotationMatrix=[1 0 0; 0 1 0; 0 0 1]
  F1 : PMIOPort  Side=Left
  F : PMIOPort  Port=2  Side=Right
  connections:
  Solid/RConn1 -- ReferenceFrame/RConn1 -- Transform/LConn1 -- Transform1/LConn1
  Transform/RConn1 -- F/RConn1
  Transform1/RConn1 -- F1/RConn1

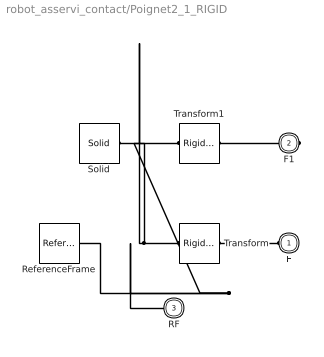
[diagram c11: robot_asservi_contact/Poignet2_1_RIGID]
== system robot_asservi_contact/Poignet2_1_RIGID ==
  ReferenceFrame : sm_lib/Frames and Transforms/Reference Frame
  Solid : sm_lib/Body Elements/Solid  InertiaType=Custom  Mass=smiData.Solid(6).mass  MassUnits=kg  CenterOfMass=smiData.Solid(6).CoM  CenterOfMassUnits=mm  MomentsOfInertia=smiData.Solid(6).MoI  MomentsOfInertiaUnits=kg*mm^2  ProductsOfInertia=smiData.Solid(6).PoI  ProductsOfInertiaUnits=kg*mm^2  DensityBased=on  Density=1000  DensityUnits=kg/m^3  DoExposeReferenceFrame=on  SerializedFrames=<Frames/>  GraphicType=FromGeometry  MarkerShape=Sphere  MarkerSize=10  GraphicVisPropType=SimpleVisualProperties  GraphicDiffuseColor=[1.0 0.0 1.0]  GraphicSpecularColor=[0.5 0.5 0.5 1.0]  GraphicAmbientColor=[0.15 0.15 0.15 1.0]  GraphicEmissiveColor=[0.0 0.0 0.0 1.0]  GraphicShininess=75  GraphicOpacity=smiData.Solid(6).opacity  GeometryShape=FromFile  RectangleSize=[1 1]  RectangleSizeUnits=m  BrickDimensions=[1 1 1]  BrickDimensionUnits=m  CylinderRadius=1  CylinderRadiusUnits=m  CylinderLength=1  CylinderLengthUnits=m  SphereRadius=1  SphereRadiusUnits=m  EllipsoidRadii=[1 1 1]  EllipsoidRadiiUnits=m  ExtrusionCrossSection=[1 1; -1 1; -1 -1; 1 -1]  ExtrusionCrossSectionUnits=m  ExtrusionLength=1  ExtrusionLengthUnits=m  PolygonNumSides=3  PolygonOuterRadius=1  PolygonOuterRadiusUnits=m  ExtGeomFileType=STL  ExtGeomFileName=Poignet2_Défaut_sldprt.STL  ExtGeomFileUnits=mm  RevolutionCrossSection=[1 1; 1 -1; 2 -1; 2 1]  RevolutionCrossSectionUnits=m  RevolutionExtent=Full  RevolutionAngle=180  RevolutionAngleUnits=deg
  Transform : sm_lib/Frames and Transforms/Rigid Transform  TranslationMethod=Cartesian  TranslationStandardOffset=0  TranslationLengthUnit=mm  TranslationStandardAxis=+Z  TranslationCartesianOffset=smiData.RigidTransform(2).translation  TranslationROffset=0  TranslationROffsetUnits=m  TranslationZOffset=0  TranslationZOffsetUnits=m  TranslationThetaOffset=0  TranslationThetaOffsetUnits=deg  RotationMethod=ArbitraryAxis  RotationAngleUnits=rad  RotationStandardAxis=+Z  RotationAngle=smiData.RigidTransform(2).angle  RotationArbitraryAxis=smiData.RigidTransform(2).axis  FollAlignAxisA=+X  BaseAlignAxisA=+Y  FollAlignAxisB=+Y  BaseAlignAxisB=+Z  RotationSequenceAxes=FollowerAxes  RotationSequence=XYX  RotationSequenceAngles=[0 0 0]  RotationSequenceAnglesUnits=deg  RotationMatrix=[1 0 0; 0 1 0; 0 0 1]
  Transform1 : sm_lib/Frames and Transforms/Rigid Transform  TranslationMethod=Cartesian  TranslationStandardOffset=0  TranslationLengthUnit=mm  TranslationStandardAxis=+Z  TranslationCartesianOffset=smiData.RigidTransform(5).translation  TranslationROffset=0  TranslationROffsetUnits=m  TranslationZOffset=0  TranslationZOffsetUnits=m  TranslationThetaOffset=0  TranslationThetaOffsetUnits=deg  RotationMethod=ArbitraryAxis  RotationAngleUnits=rad  RotationStandardAxis=+Z  RotationAngle=smiData.RigidTransform(5).angle  RotationArbitraryAxis=smiData.RigidTransform(5).axis  FollAlignAxisA=+X  BaseAlignAxisA=+Y  FollAlignAxisB=+Y  BaseAlignAxisB=+Z  RotationSequenceAxes=FollowerAxes  RotationSequence=XYX  RotationSequenceAngles=[0 0 0]  RotationSequenceAnglesUnits=deg  RotationMatrix=[1 0 0; 0 1 0; 0 0 1]
  F : PMIOPort  Side=Left
  F1 : PMIOPort  Port=2  Side=Right
  RF : PMIOPort  Port=3  Side=Left
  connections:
  Solid/RConn1 -- RF/RConn1 -- ReferenceFrame/RConn1 -- Transform/LConn1 -- Transform1/LConn1
  Transform/RConn1 -- F/RConn1
  Transform1/RConn1 -- F1/RConn1
